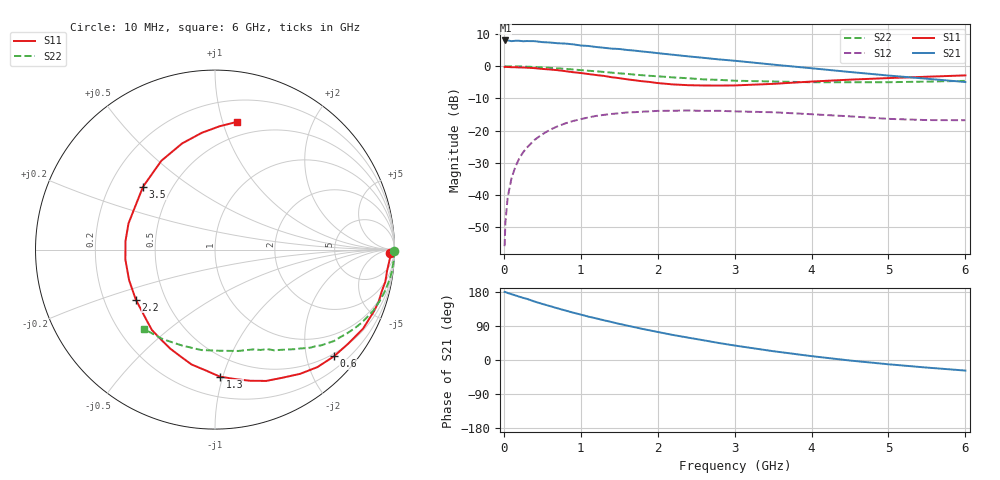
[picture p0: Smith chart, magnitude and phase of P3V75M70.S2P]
! SIEMENS Small Signal Semiconductors
! BFP181
! Si NPN RF Bipolar Junction Transistor in SOT143
! VCE = 0.75 V  IC = 0.7 mA
! Common Emitter S-Parameters:  March  1996
# GHz  S  MA  R  50
!  f  S11  S21  S12  S22
! GHz  MAG  ANG  MAG  ANG  MAG  ANG  MAG  ANG
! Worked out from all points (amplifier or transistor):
!   36 points, 10 MHz to 6 GHz, reference 50 ohm
!   highest |S21| = 8.0 dB at 20 MHz (marker M1)
!   |S21| within 3 dB of that: start of sweep to 1.623 GHz
!   unconditionally stable (mu >= 1): 3.177 GHz to end of sweep
!   at 250 MHz: K = 0.09, MSG = 17.3 dB, |S12| = -26.8 dB
!   at 1.4 GHz: K = 0.49, MSG = 10.2 dB, |S12| = -14.8 dB
!   at 6 GHz: K = 1.50, MAG = 1.7 dB, |S12| = -16.8 dB
!   S11 on the Smith chart (normalised r, x): 10 MHz: 52, -33; 600 MHz: 0.44, -2.55; 1.3 GHz: 0.34, -0.98; 2.2 GHz: 0.34, -0.26; 3.5 GHz: 0.34, +0.34; 6 GHz: 0.38, +1.11
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0.01  0.9727 -1.0  2.483 179.7  0.0016 82.1  0.9984 -0.3
0.02  0.9802 -1.5  2.517 179.4  0.0037 89.1  0.9967 -0.7
0.05  0.974 -3.5  2.516 176.9  0.0092 89.5  0.9975 -1.8
0.1  0.9659 -7.1  2.455 173.7  0.0183 83.6  0.9967 -3.6
0.2  0.9576 -14.1  2.487 167.1  0.0369 80.5  0.9923 -7.3
0.3  0.9498 -21.3  2.464 161.4  0.0545 75.5  0.9839 -10.7
0.4  0.9352 -28.1  2.453 154.2  0.0719 70.5  0.9735 -14.2
0.6  0.8908 -41.8  2.338 142.2  0.1031 61.1  0.946 -20.9
0.8  0.8395 -55.5  2.25 130.6  0.1296 52.4  0.911 -26.8
0.9  0.8081 -61.9  2.19 125.0  0.1411 48.0  0.8902 -29.8
1.1  0.7571 -74.9  2.066 114.4  0.1602 40.5  0.8512 -35.0
1.3  0.7084 -87.8  1.937 104.9  0.1756 33.4  0.8152 -39.8
1.5  0.6534 -101.5  1.855 95.4  0.1859 27.3  0.7761 -43.9
1.8  0.5846 -120.9  1.694 82.1  0.1968 19.5  0.7257 -49.4
2.2  0.5218 -147.8  1.509 66.0  0.2035 9.7  0.6709 -56.3
2.8  0.501 174.7  1.276 44.7  0.2031 -1.4  0.6145 -65.5
3  0.5036 163.1  1.218 38.2  0.1989 -4.9  0.596 -68.9
3.5  0.5326 138.8  1.061 23.3  0.1929 -11.0  0.5795 -77.0
4  0.5783 121.1  0.931 10.2  0.1797 -16.0  0.5646 -86.8
4.5  0.6193 107.2  0.814 -1.4  0.1665 -19.8  0.5649 -97.7
5.5  0.6875 87.9  0.64 -20.0  0.1458 -17.6  0.5773 -120.1
6  0.7212 80.4  0.569 -27.9  0.145 -15.1  0.5931 -131.5
